ORGANIZATION_BLOCK MAIN:OB1
TITLE=Ciclo automatico A+/B+/C+/(A- B- C-) con cilindri a doppio
//effetto e tre valvole monostabili.
//Simulatore: 15
//Versione 1.0
//Data: 28/02/2002
//------------- DESCRIZIONE DEL CONTROLLO ---------------------
// L'esempio utilizza tre cilindri (A, B, C) a doppio effetto e tre
// elettrovalvole 5/2 monostabili (1V1, 2V1, 3V1).
// Una valvola 3/2 monostabile 0V permette la distribuzione dell'aria al
// circuito.
// Un Pulsante SB1 da inizio al ciclo ripetitivo che può essere
// interrotto dal pulsante di Stop SB3.
// Il pulsante SB2 da invece inizio ad un solo ciclo completo.
// Due lampade HL1, HL2 e HL3 indicano rispettivamente: la presenza
// dell'aria, il modo di funzionamento con ciclo ripetitivo e
// l'intervento del circuito di sicurezza esterna.
// I collegamenti agli ingressi del PLC sono:
// - Il selettore SB6 per il comando dell'aria compressa;
// - Il pulsante di arresto ciclo SB3;
// - Il pulsante di avvio ciclo in semiautomatico SB2;
// - il pulsante di avvio ciclo automatico SB1;
// - i fine corsa magnetici per il controllo della posizione
//   dei pistoni dei tre cilindri;
// Due lampade segnalano rispettivamente:
// - HL1 Presenza aria
// - HL2 Ciclo ripetitivo attivo
//

BEGIN
NETWORK 1 //Azinamento elettrovalvola Aria
//
//COMMENTI DEL SEGMENTO
//
LD I0.6
= Q0.0

NETWORK 2 //Memoria ciclo automatico
//
LD I0.7
O M0.0
A I1.1
= M0.0

NETWORK 3 //Corsa + Pistone A
//
LD M0.0
O I1.0
A I0.0
A I0.2
A I0.4
O Q0.1
AN I0.5
AN M1.0
= Q0.1

NETWORK 4 //Corsa + Pistone B
//
LDN I0.5
A I0.1
AN I0.0
= Q0.2

NETWORK 5 //Corsa + Pistone C
//
LDN I0.5
A I0.3
AN I0.2
= Q0.3

NETWORK 6 //Gestione merker ripartenza
//
LD I0.5
LD M1.0
A I1.0
OLD
= M1.0

NETWORK 7 //Lampada presenza aria
//
LD Q0.0
= Q0.4

NETWORK 8 //Lampada ciclo automatico
//
LD M0.0
= Q0.5

END_ORGANIZATION_BLOCK

